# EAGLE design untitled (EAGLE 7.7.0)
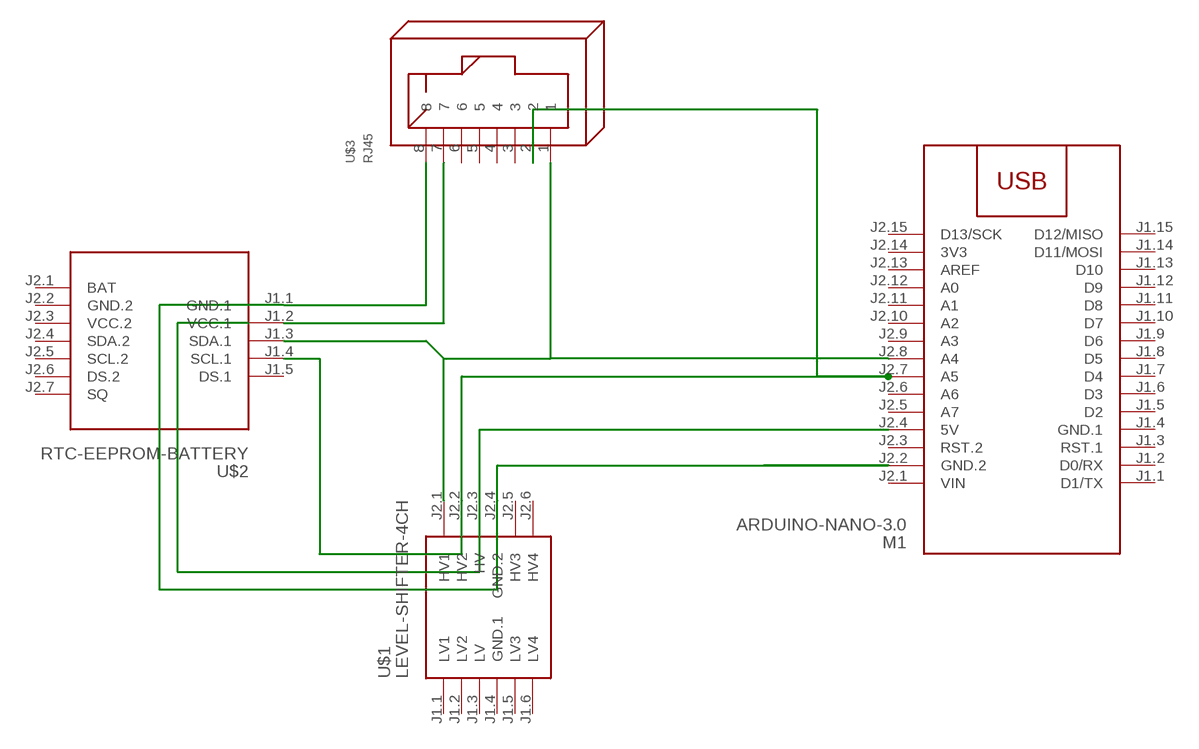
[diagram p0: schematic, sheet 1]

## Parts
M1  ARDUINO-NANO-3.0  [ARDUINO-NANO-3.0]
U$1  LEVEL-SHIFTER-4CH  [LEVEL-SHIFTER-4CH]
U$2  RTC-EEPROM-BATTERY  [RTC-EEPROM-BATTERY]
U$3  RJ45  [RJ45]

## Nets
N$1: M1.J2.4(5V) U$1.J2.3(HV)
N$2: M1.J2.2(GND.2) U$1.J2.4(GND.2) U$2.J1.1(GND.1) U$3.8
N$3: M1.J2.7(A5) U$1.J2.2(HV2) U$2.J1.4(SCL.1) U$3.2
N$4: M1.J2.8(A4) U$1.J2.1(HV1) U$2.J1.3(SDA.1) U$3.1
N$8: U$2.J1.2(VCC.1) U$3.7
Unconnected: M1.J1.1(D1/TX) M1.J1.2(D0/RX) M1.J1.3(RST.1) M1.J1.5(D2) M1.J1.6(D3) M1.J1.7(D4) M1.J1.8(D5) M1.J1.9(D6) M1.J1.10(D7) M1.J1.11(D8) M1.J1.12(D9) M1.J1.13(D10) M1.J1.14(D11/MOSI) M1.J1.15(D12/MISO) M1.J2.3(RST.2) M1.J2.5(A7) M1.J2.6(A6) M1.J2.9(A3) M1.J2.10(A2) M1.J2.11(A1) M1.J2.12(A0) M1.J2.13(AREF) M1.J2.15(D13/SCK) U$1.J1.1(LV1) U$1.J1.2(LV2) U$1.J1.5(LV3) U$1.J1.6(LV4) U$1.J2.5(HV3) U$1.J2.6(HV4) U$2.J1.5(DS.1) U$2.J2.1(BAT) U$2.J2.4(SDA.2) U$2.J2.5(SCL.2) U$2.J2.6(DS.2) U$2.J2.7(SQ) U$3.3 U$3.4 U$3.5 U$3.6

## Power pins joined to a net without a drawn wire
3V3: M1.J2.14(3V3)
GND.1: M1.J1.4(GND.1) U$1.J1.4(GND.1)
GND.2: U$2.J2.2(GND.2)
LV: U$1.J1.3(LV)
VCC.2: U$2.J2.3(VCC.2)
VIN: M1.J2.1(VIN)

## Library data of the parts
M1 = diy-modules:ARDUINO-NANO-3.0: Arduino Nano 3.0 and compatible devices More details available here: https://www.arduino.cc/en/Main/ArduinoBoardNano Click here to find device on ebay.com
U$1 = diy-modules:LEVEL-SHIFTER-4CH: 4-Channel Bi-Directional Logic Level Converter based on BSS128 transistors Click here to find device on ebay.com
U$2 = diy-modules:RTC-EEPROM-BATTERY: RTC Module with Battery and EEPROM based on DS1307 and AT24C32 chips More details available here: http://henrysbench.capnfatz.com/henrys-bench/arduino-sensors-and-input/arduino-tiny-rtc-d1307-tutorial/ Click here to find device on ebay.com
U$3 = con-rj:RJ45: RJ45 RJ45 jacks side mounted http://www.tycoelectronics.com

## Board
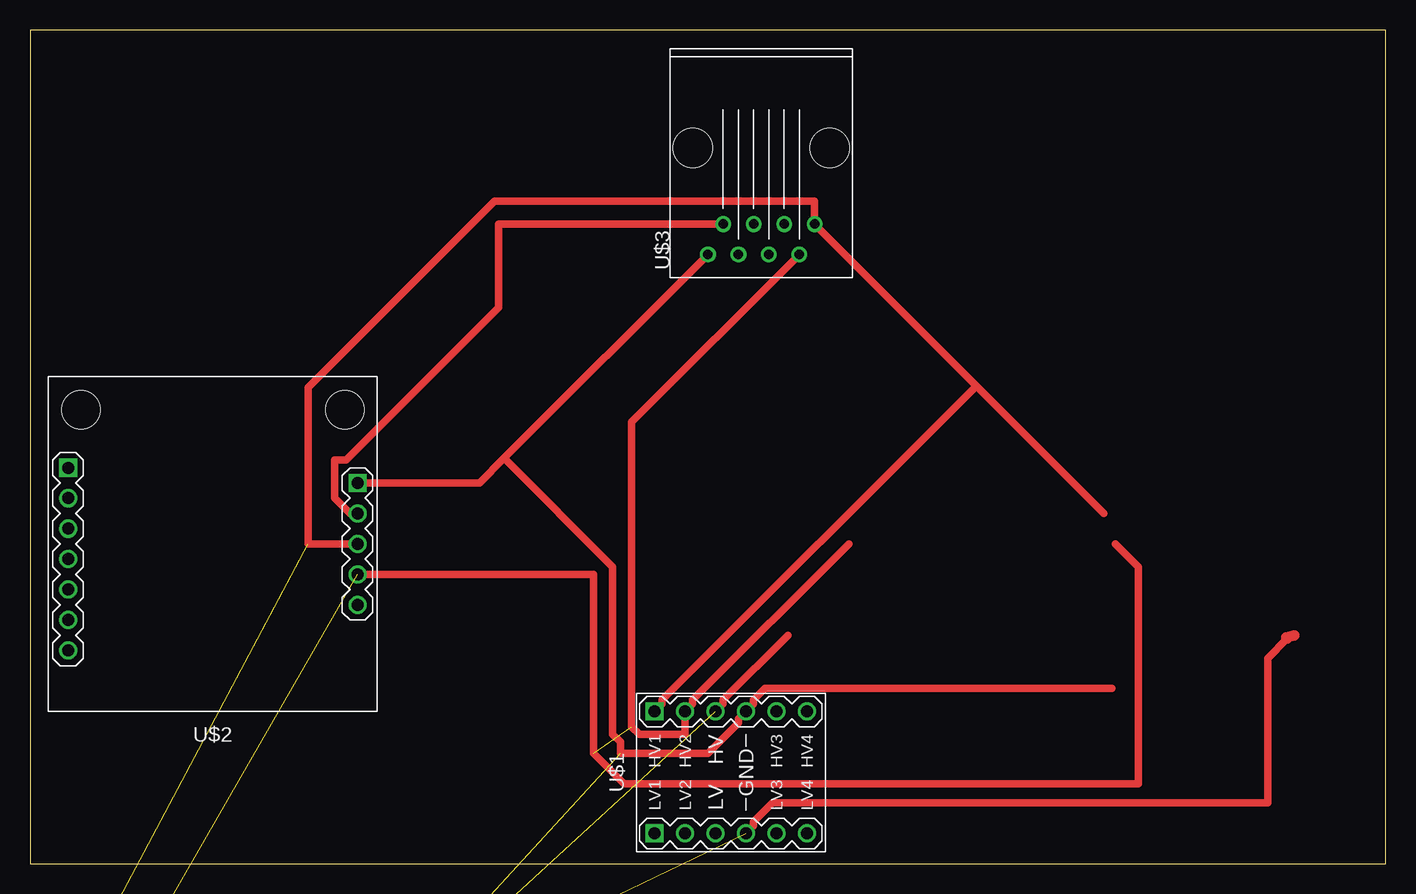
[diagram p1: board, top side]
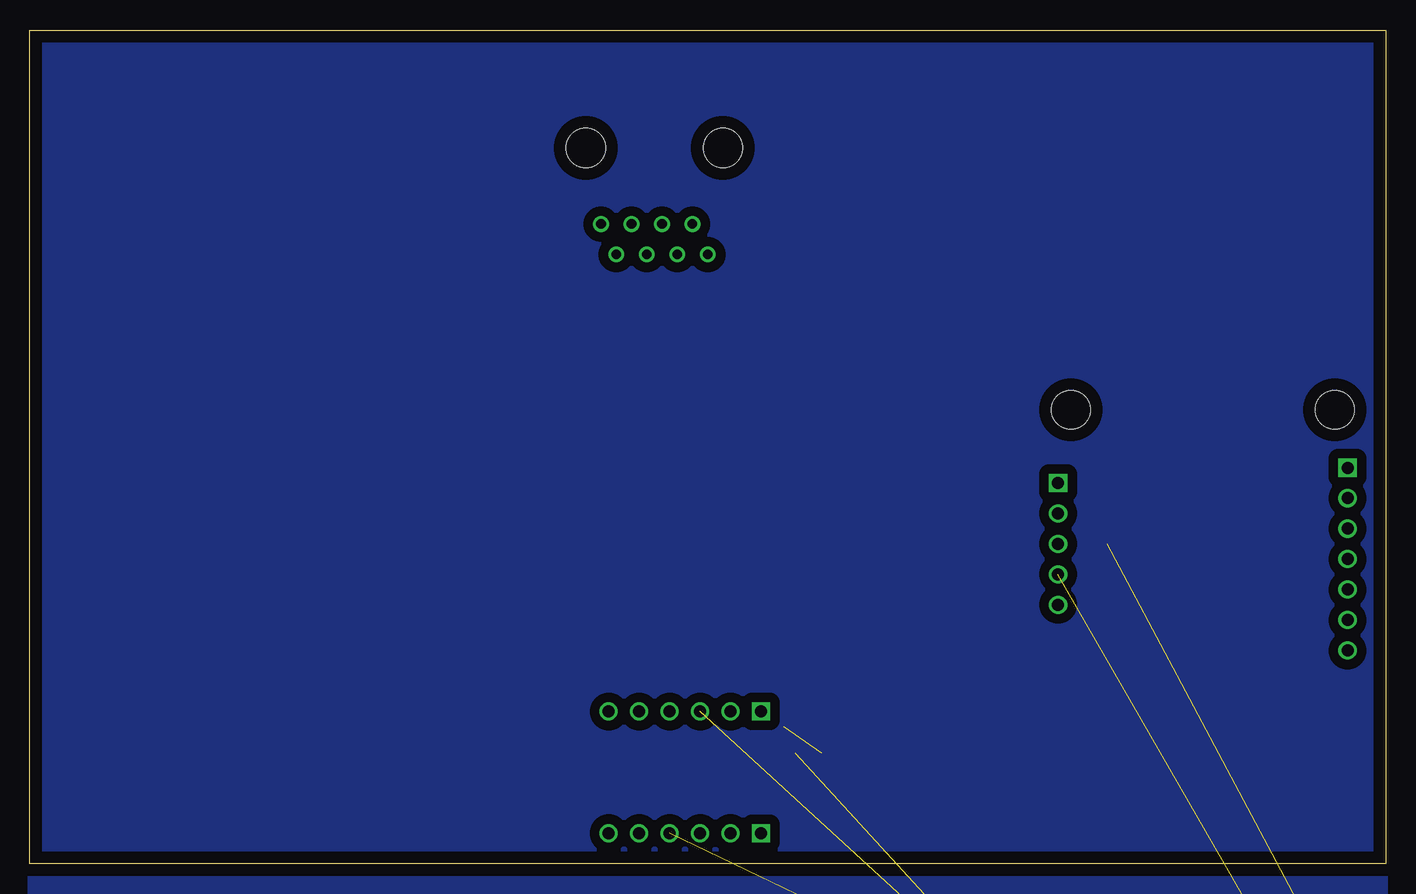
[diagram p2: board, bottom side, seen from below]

Size 113.01 x 69.52 mm. Coordinates in mm from the lower left corner, seen from the top.
Outline: 0,0 113.01,0 113.01,69.52 0,69.52 0,0
Copper layers (1*16): Top 0.035mm / dielectric 1.5mm / Bottom 0.035mm
Design rules "default *": minimum track width 35mil, minimum drill 24mil, track to track 32mil, track to pad 32mil, pad to pad 32mil, via to via 32mil, smd to smd 32mil, copper to edge 40mil, drill to drill 8mil, minimum pad ring 10mil, minimum via ring 8mil, stop-mask expansion 4mil, vias tented up to drill 0mil, thermal gap 10mil

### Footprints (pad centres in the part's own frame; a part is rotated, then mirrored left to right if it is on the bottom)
ARDUINO-NANO-3.0 = drill 1 square: J1.1 17.78,7.62 | drill 1: J1.2 15.24,7.62; J1.3 12.7,7.62; J1.4 10.16,7.62; J1.5 7.62,7.62; J1.6 5.08,7.62; J1.7 2.54,7.62; J1.8 0,7.62; J1.9 -2.54,7.62; J1.10 -5.08,7.62; J1.11 -7.62,7.62; J1.12 -10.16,7.62; J1.13 -12.7,7.62; J1.14 -15.24,7.62; J1.15 -17.78,7.62; J2.1 17.78,-7.62; J2.2 15.24,-7.62; J2.3 12.7,-7.62; J2.4 10.16,-7.62; J2.5 7.62,-7.62; J2.6 5.08,-7.62; J2.7 2.54,-7.62; J2.8 0,-7.62; J2.9 -2.54,-7.62; J2.10 -5.08,-7.62; J2.11 -7.62,-7.62; J2.12 -10.16,-7.62; J2.13 -12.7,-7.62; J2.14 -15.24,-7.62; J2.15 -17.78,-7.62 | hole 1.651: -20.32,7.62; -20.32,-7.62; 20.32,-7.62; 20.32,7.62
LEVEL-SHIFTER-4CH = drill 1 square: J1.1 -5.08,6.35; J2.1 5.08,6.35 | drill 1: J1.2 -5.08,3.81; J1.3 -5.08,1.27; J1.4 -5.08,-1.27; J1.5 -5.08,-3.81; J1.6 -5.08,-6.35; J2.2 5.08,3.81; J2.3 5.08,1.27; J2.4 5.08,-1.27; J2.5 5.08,-3.81; J2.6 5.08,-6.35
RTC-EEPROM-BATTERY = drill 1 square: J1.1 -12.065,-5.08; J2.1 12.065,-6.35 | drill 1: J1.2 -12.065,-2.54; J1.3 -12.065,0; J1.4 -12.065,2.54; J1.5 -12.065,5.08; J2.2 12.065,-3.81; J2.3 12.065,-1.27; J2.4 12.065,1.27; J2.5 12.065,3.81; J2.6 12.065,6.35; J2.7 12.065,8.89 | hole 3.2: -11,-11.176; 11,-11.176
RJ45 = drill 0.8: 1 -6.35,-4.445; 2 -8.89,-3.175; 3 -6.35,-1.905; 4 -8.89,-0.635; 5 -6.35,0.635; 6 -8.89,1.905; 7 -6.35,3.175; 8 -8.89,4.445 | hole 3.25: 0,-5.715; 0,5.715

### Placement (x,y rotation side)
M1  not placed on the board
U$1  58.42,7.62 90 top
U$2  15.24,26.67 180 top
U$3  60.96,59.69 90 top

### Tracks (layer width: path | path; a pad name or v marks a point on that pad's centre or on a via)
GND.1  (1 unrouted)
  Top 0.635: U$1.J1.4 60.33,3.17 60.33,3.49 61.91,5.08 103.19,5.08 103.19,17.14 104.83,18.78 105.09,19.05
  Top 0.889: 105.41,19.05 104.72,18.88 104.83,18.78
N$1  (1 unrouted)
  Top 0.635: U$1.J2.3 57.78,13.33 57.78,13.65 63.18,19.05
N$2  (1 unrouted)
  Top 0.635: 90.17,14.6 61.28,14.6 60.33,13.65 60.33,13.33 U$1.J2.4 59.05,12.06 59.05,11.75 56.52,9.21 49.21,9.21 49.21,10.16 48.58,10.79 48.58,24.76 39.53,33.81 | 39.53,33.81 37.47,31.75 U$2.J1.1 | 39.53,33.81 U$3.8
N$3  (2 unrouted)
  Top 0.635: U$3.2 50.17,36.83 50.17,11.43 50.8,10.79 54.61,10.79 U$1.J2.2 55.24,13.33 55.24,13.65 68.26,26.67 | U$2.J1.4 46.99,24.13 46.99,9.21 49.53,6.67 92.39,6.67 92.39,24.76 90.49,26.67
N$4  (1 unrouted)
  Top 0.635: 89.53,29.21 78.9,39.85 | 78.9,39.85 U$3.1 65.41,55.24 38.73,55.24 23.18,39.69 23.18,26.67 U$2.J1.3 | U$1.J2.1 52.7,13.33 52.7,13.65 78.9,39.85
N$5
  pour Bottom: 0,68.58 113.03,68.58 113.03,-19.05 0,-19.05
N$8
  Top 0.635: U$3.7 39.05,53.34 39.05,46.35 26.35,33.65 25.4,33.65 25.4,30.48 26.67,29.21 U$2.J1.2

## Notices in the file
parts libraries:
diy-modules: Released under the Creative Commons Attribution 4.0 International License: http://creativecommons.org/licenses/by/4.0
